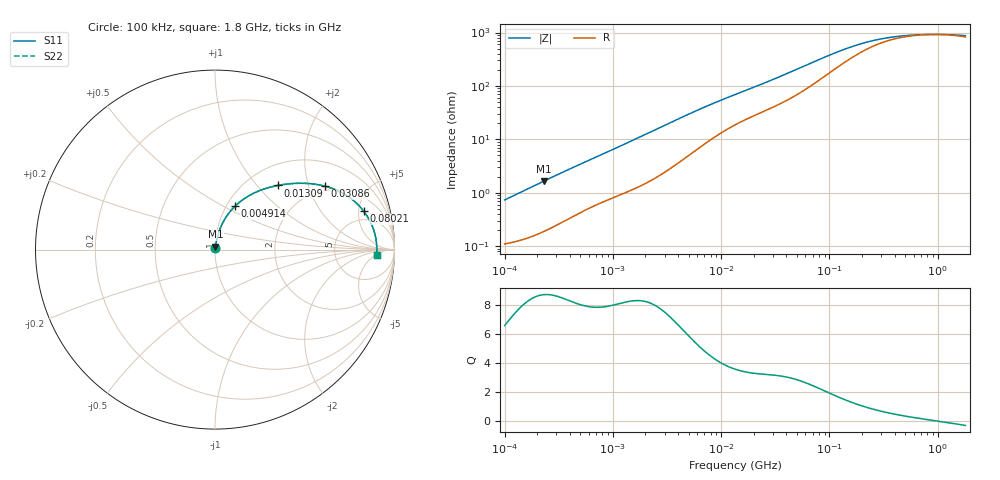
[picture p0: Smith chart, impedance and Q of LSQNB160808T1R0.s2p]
! LSQNB160808T1R0  S-PARAMETER MODEL  ( General Type )
! Model Generated by TAIYO YUDEN Corporation (http://www.ty-top.com)
! Version 2.0
! TAIYO YUDEN Control No. 100810NF25SB-FKC
! Copyright(c) 2007 TAIYO YUDEN CO.,LTD. All Rights Reserved.
! Product Description (link to TY-COMPAS)
! https://ds.yuden.co.jp/TYCOMPAS/or/detail?pn=LSQNB160808T1R0M&u=M
! Products Name : Inductors
! Characteristics :
!  Inductance : 1.0 uH , SRF(min) : 100 MHz , DC Resistance(max) : 0.117 Ohm
!  Rated Current : Saturation :290 mA , Temp Rise : 770 mA (40 degC)
!  Case Size : 1.6 x 0.8 / 0.063 x 0.031 [mm/inch] , Thickness : 0.8 / 0.031 [mm/inch]
!  (Conditions: Temperature = 25 degC , DC Bias Current/Voltage = 0A / 0V)
! External Node Assignments :
!  1  o---GGG---o  2
! GND o---------o GND
! Frequency Range : 0.1MHz  -  1800MHz  [ 402 STEP ]
# MHz S RI R 50
! Freq[MHz].  S11 Real  S11 Imag  S21 Real  S21 Imag  S12 Real  S12 Imag  S22 Real  S22 Imag
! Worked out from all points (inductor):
!   401 points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, 100 kHz to 1.8 GHz, reference 50 ohm
!   read as one part in series: L = 1.15 uH near 105 kHz
!   highest Q = 8.71 at 230 kHz (marker M1), where L = 1.14 uH
!   self-resonance near 932.2 MHz
!   S11 on the Smith chart (normalised r, x): 100 kHz: 1.00, +0.01; 4.914 MHz: 1.10, +0.57; 13.09 MHz: 1.36, +1.30; 30.86 MHz: 1.82, +2.57; 80.21 MHz: 3.56, +5.70; 1.8 GHz: 18, -6
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0.1  0.00116 0.00724  0.9988 -0.00724  0.9988 -0.00724  0.00116 0.00724
0.229984  0.00215 0.0164  0.9978 -0.0164  0.9978 -0.0164  0.00215 0.0164
0.516129  0.00559 0.0348  0.9944 -0.0348  0.9944 -0.0348  0.00559 0.0348
1.277529  0.016 0.0786  0.984 -0.0786  0.984 -0.0786  0.016 0.0786
2.66389  0.0444 0.1516  0.9556 -0.1516  0.9556 -0.1516  0.0444 0.1516
4.914404  0.1128 0.243  0.8872 -0.243  0.8872 -0.243  0.1128 0.243
8.02111  0.2158 0.3143  0.7842 -0.3143  0.7842 -0.3143  0.2158 0.3143
13.09176  0.3507 0.3577  0.6493 -0.3577  0.6493 -0.3577  0.3507 0.3577
13.41641  0.3579 0.3591  0.6421 -0.3591  0.6421 -0.3591  0.3579 0.3591
20.85084  0.4911 0.3696  0.5089 -0.3696  0.5089 -0.3696  0.4911 0.3696
30.85563  0.6127 0.3534  0.3873 -0.3534  0.3873 -0.3534  0.6127 0.3534
47.95365  0.7347 0.3005  0.2653 -0.3005  0.2653 -0.3005  0.7347 0.3005
69.24595  0.8078 0.239  0.1922 -0.239  0.1922 -0.239  0.8078 0.239
80.20907  0.8288 0.2139  0.1712 -0.2139  0.1712 -0.2139  0.8288 0.2139
115.8234  0.8648 0.1563  0.1352 -0.1563  0.1352 -0.1563  0.8648 0.1563
184.4683  0.8872 0.0994  0.1128 -0.0994  0.1128 -0.0994  0.8872 0.0994
259.9299  0.8949 0.0685  0.1051 -0.0685  0.1051 -0.0685  0.8949 0.0685
357.3983  0.8986 0.0464  0.1014 -0.0464  0.1014 -0.0464  0.8986 0.0464
516.0898  0.9007 0.0262  0.0993 -0.0262  0.0993 -0.0262  0.9007 0.0262
763.7235  0.9017 0.00841  0.0983 -0.00841  0.0983 -0.00841  0.9017 0.00841
1186.925  0.9018 -0.0102  0.0982 0.0102  0.0982 0.0102  0.9018 -0.0102
1800  0.901 -0.0296  0.099 0.0296  0.099 0.0296  0.901 -0.0296
